(* Sampled values subscriber *)
{attribute 'no_assign'}
FUNCTION_BLOCK FB_IED_MUnn_MSVCB02SvSubscriber IMPLEMENTS I_GseLinkStatusEventSink, I_GseSvUpdateEventSink
VAR_INPUT
	fbAdapter: FB_GseAdapterClass := (ipLinkStatus:=THIS^); (* GSE network adapter *)
END_VAR
VAR_OUTPUT
	fbApdu1: FB_SVRXAPDU_IED_MUnn_LLN0_MSVCB02 := (ipUpdate:=THIS^); (* SV subscriber APDU *)
	(*
	fbApdu2: FB_SVRXAPDU_...
	...
	fbApduN: FB_SVRXAPDU_...
	*)
	RxBuffer1: ST_SVBUFFER_IED_MUnn_LLN0_MSVCB02; (* SV data buffer *)
	(*
	RxBuffer2: ST_SVBUFFER_...
	...
	RxBufferN: ST_SVBUFFER_...
	*)
END_VAR
VAR
	eLinkStatus: E_GseLinkStatus; (* Network adapter link status *)
	bSuccess: BOOL;
	ipError: I_ServiceErrorClass;
	bSubscribe: BOOL := TRUE; (* Rising edge enables subscriber SvCB's *)
	bUnsubscribe: BOOL; (* Rising edge disables subscriber SvCB's *)
	
	bSynch: BOOL; (* If TRUE => sample counter is 0 *)
	nSynch: UDINT; (* Increments every time sample counter is 0 *)
	nSmpCnt: UINT; (* Sample counter *)
	eSmpSynch: E_GseSvSmpSynch := E_GseSvSmpSynch.None; (* Synchronization type: 0..2 *)
	tRefrTm: T_UtcTime; (* Sample refresh time stamp (optional) *)
	bSimulation: BOOL; (* SV ethernet header simulation flag *)
END_VAR

bSuccess:= fbAdapter.Execute(ipError=>ipError); (* Execute network adapter *)

IF bSubscribe THEN (* Enable subscriber SvCB's *)
	bSubscribe:= FALSE;
	bSuccess:= fbIED.IEDMUnn.LLN0.MSVCB02.Subscriber.Enable(ipAdapter:=fbAdapter, ipApdu:=fbApdu1, ipError=>ipError);
ELSIF bUnsubscribe THEN (* Disable subscriber SvCB's *)
	bUnsubscribe:= FALSE;
	bSuccess:= fbIED.IEDMUnn.LLN0.MSVCB02.Subscriber.Disable(ipError=>ipError);
ELSE (* Execute subscriber SvCB's *)
	bSuccess:= fbIED.IEDMUnn.LLN0.MSVCB02.Subscriber.Execute(ipError=>ipError);
END_IF

{attribute 'analysis' := '-33'}
(* This method is called every time the network adapter link status changes *)
METHOD FINAL OnLinkStatusChange
VAR_INPUT
	ipAdapter: I_GseAdapterClass; (* Interface pointer of the network adapter reporting link status change *)
	eStatus: E_GseLinkStatus; (* New (changed) link status *)
END_VAR
VAR
END_VAR
eLinkStatus:= eStatus;
END_METHOD

{attribute 'analysis' := '-33'}
(* This method receives SV APDU update event notification *)
METHOD FINAL OnSvUpdate
VAR_INPUT
	ipAdapter: I_GseAdapterClass; (* Network adapter interface pointer *)
	ipApdu: I_GseSvApduClass; (* APDU object interface pointer *)
END_VAR
VAR
	index: UINT; (* Temp. variable *)
END_VAR
(* Hint: The time stamp will only be sent if "RefreshTime" parameter in the "OptFlds" of the SV publisher control block is set to TRUE *)

(* Find the updated APDU object and process the received data *)
IF fbApdu1.Equals(ipOther:=ipApdu) THEN

	bSimulation:= fbApdu1.bSimulation; (* Get SV ethernet header simulation flag *)
	FOR index:=0 TO cOversampleFactor_IED_MUnn_LLN0_MSVCB02_Asdu1-1 BY 1 DO

		nSmpCnt:= fbApdu1.RxData.Asdu1.nSmpCnt[index]; (* Get sample counter *)
		eSmpSynch:= fbApdu1.RxData.Asdu1.eSmpSynch[index]; (* Get synchronization type: 0..2 *)
		tRefrTm:= fbApdu1.RxData.Asdu1.tRefrTm[index]; (* Get sample refresh time stamp (optional) *)
		IF nSmpCnt = 0 THEN
			bSynch:= TRUE;
			nSynch:= nSynch + 1;
		END_IF

		RxBuffer1.IED_MUnn_InnATCTR1_AmpSv_instMag_i[RxBuffer1.index]:= fbApdu1.RxData.Asdu1.IED_MUnn_InnATCTR1_AmpSv_instMag_i[index];
		RxBuffer1.IED_MUnn_InnATCTR1_AmpSv_q[RxBuffer1.index]:= fbApdu1.RxData.Asdu1.IED_MUnn_InnATCTR1_AmpSv_q[index];
		RxBuffer1.IED_MUnn_InnBTCTR2_AmpSv_instMag_i[RxBuffer1.index]:= fbApdu1.RxData.Asdu1.IED_MUnn_InnBTCTR2_AmpSv_instMag_i[index];
		RxBuffer1.IED_MUnn_InnBTCTR2_AmpSv_q[RxBuffer1.index]:= fbApdu1.RxData.Asdu1.IED_MUnn_InnBTCTR2_AmpSv_q[index];
		RxBuffer1.IED_MUnn_InnCTCTR3_AmpSv_instMag_i[RxBuffer1.index]:= fbApdu1.RxData.Asdu1.IED_MUnn_InnCTCTR3_AmpSv_instMag_i[index];
		RxBuffer1.IED_MUnn_InnCTCTR3_AmpSv_q[RxBuffer1.index]:= fbApdu1.RxData.Asdu1.IED_MUnn_InnCTCTR3_AmpSv_q[index];
		RxBuffer1.IED_MUnn_InnNTCTR4_AmpSv_instMag_i[RxBuffer1.index]:= fbApdu1.RxData.Asdu1.IED_MUnn_InnNTCTR4_AmpSv_instMag_i[index];
		RxBuffer1.IED_MUnn_InnNTCTR4_AmpSv_q[RxBuffer1.index]:= fbApdu1.RxData.Asdu1.IED_MUnn_InnNTCTR4_AmpSv_q[index];
		RxBuffer1.IED_MUnn_UnnATVTR1_VolSv_instMag_i[RxBuffer1.index]:= fbApdu1.RxData.Asdu1.IED_MUnn_UnnATVTR1_VolSv_instMag_i[index];
		RxBuffer1.IED_MUnn_UnnATVTR1_VolSv_q[RxBuffer1.index]:= fbApdu1.RxData.Asdu1.IED_MUnn_UnnATVTR1_VolSv_q[index];
		RxBuffer1.IED_MUnn_UnnBTVTR2_VolSv_instMag_i[RxBuffer1.index]:= fbApdu1.RxData.Asdu1.IED_MUnn_UnnBTVTR2_VolSv_instMag_i[index];
		RxBuffer1.IED_MUnn_UnnBTVTR2_VolSv_q[RxBuffer1.index]:= fbApdu1.RxData.Asdu1.IED_MUnn_UnnBTVTR2_VolSv_q[index];
		RxBuffer1.IED_MUnn_UnnCTVTR3_VolSv_instMag_i[RxBuffer1.index]:= fbApdu1.RxData.Asdu1.IED_MUnn_UnnCTVTR3_VolSv_instMag_i[index];
		RxBuffer1.IED_MUnn_UnnCTVTR3_VolSv_q[RxBuffer1.index]:= fbApdu1.RxData.Asdu1.IED_MUnn_UnnCTVTR3_VolSv_q[index];
		RxBuffer1.IED_MUnn_UnnNTVTR4_VolSv_instMag_i[RxBuffer1.index]:= fbApdu1.RxData.Asdu1.IED_MUnn_UnnNTVTR4_VolSv_instMag_i[index];
		RxBuffer1.IED_MUnn_UnnNTVTR4_VolSv_q[RxBuffer1.index]:= fbApdu1.RxData.Asdu1.IED_MUnn_UnnNTVTR4_VolSv_q[index];

		RxBuffer1.index:= SEL(RxBuffer1.index >= cArrayBufferSize_IED_MUnn_LLN0_MSVCB02_Asdu1-1, RxBuffer1.index + 1, 0);

	END_FOR

	(*
	ELSIF fbApdu2.Equals(ipOther:=ipApdu) THEN
		;
	ELSIF fbApduN.Equals(ipOther:=ipApdu) THEN
		;
	*)
END_IF
END_METHOD

END_FUNCTION_BLOCK
